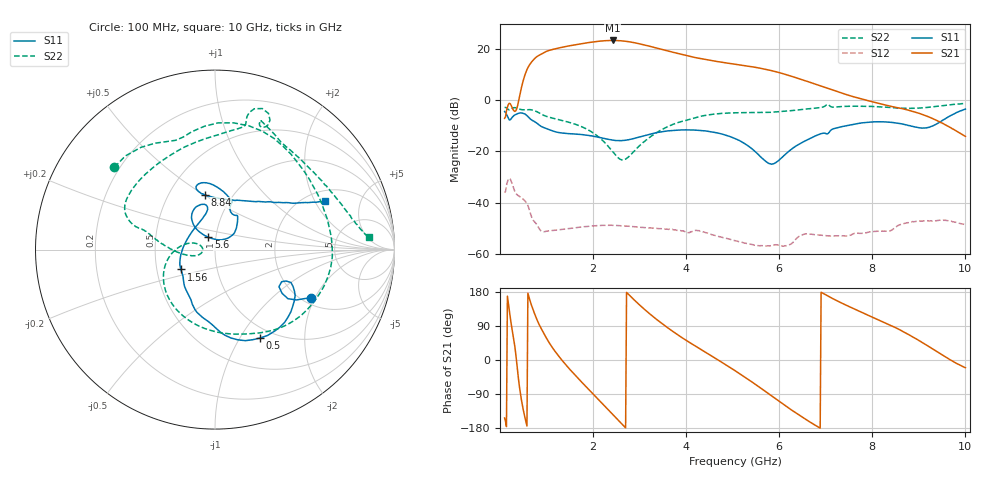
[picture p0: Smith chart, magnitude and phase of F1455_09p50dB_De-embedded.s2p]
! Integrated Device Technology
! Corporate Headquarters
! 6024 Silver Creek Valley Road
! San Jose, CA 95138  USA
! Phone:  1-408-284-8200
! Toll Free:  1-800-223-1366
! Webpage:  http://www.idt.com/
! Timing and RF Division
! 515 Groton Road, Suite 102
! Westford, MA 01886-6024
! Device:  F1455
! Description: 6-bit 0.5 dB Transmit Variable Gain Amplifier
! Frequency:  1400.0 -  2300.00 MHz
! Package:  6x6 mm Thin QFN Plastic Package: 28 pin
! State:  19
! Atten State:  9.5 dB
! Voltage:  +5.00 Volts
! Current:  217.652 mA
! Data:  The device was measured on a the F1455 evaluation board which has
!  individual transmission lines to the RF pins.  Data was collected
!  using a calibrated network analyzer.  The evaluation board was
!  de-embedded using a TRL calibration technique.
!  The reference plane is the edge of the package pin.
!  Pin  1 = CSb
!  Pin  2 = DATA
!  Pin  3 = CLK
!  Pin  4 = RSET
!  Pin  5 = GND
!  Pin  6 = RFIN  = Port 1
!  Pin  7 = GND
!  Pin  8 = NC
!  Pin  9 = NC
!  Pin 10 = NC
!  Pin 11 = NC
!  Pin 12 = NC
!  Pin 13 = NC
!  Pin 14 = /STBY
!  Pin 15 = GND
!  Pin 16 = RFOUT  = Port 2
!  Pin 17 = GND
!  Pin 18 = NC
!  Pin 19 = NC
!  Pin 20 = NC
!  Pin 21 = GND
!  Pin 22 = NC
!  Pin 23 = GND
!  Pin 24 = NC
!  Pin 25 = NC
!  Pin 26 = NC
!  Pin 27 = GND
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# GHz S dB R 50
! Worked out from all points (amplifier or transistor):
!   496 points, 100 MHz to 10 GHz, reference 50 ohm
!   highest |S21| = 23.3 dB at 2.42 GHz (marker M1)
!   |S21| within 3 dB of that: 1.25 GHz to 3.375 GHz (2.125 GHz wide, 91.9 % of centre)
!   unconditionally stable (mu >= 1): start of sweep to end of sweep
!   at 1.74 GHz: K = 10.24, MAG = 22.7 dB, |S12| = -49.6 dB
!   at 5.06 GHz: K = 36.17, MAG = 15.9 dB, |S12| = -54.9 dB
!   at 10 GHz: K = 96.42, MAG = -5.6 dB, |S12| = -48.6 dB
!   S11 on the Smith chart (normalised r, x): 100 MHz: 2.22, -1.88; 500 MHz: 0.87, -1.23; 1.56 GHz: 0.67, -0.15; 5.6 GHz: 0.92, +0.13; 8.84 GHz: 0.75, +0.50; 10 GHz: 2.46, +2.43
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0.1  -4.42 -26.7  -7.07 -152.9  -36.14 44.7  -2.80 140.7
0.38  -5.24 -39.4  -2.09 -30.2  -37.11 -111.5  -3.23 56.6
0.5  -5.15 -62.9  7.67 -130.9  -38.70 -149.6  -3.74 28.2
0.7  -7.94 -95.6  15.37 136.6  -46.45 146.9  -3.87 -18.6
0.82  -9.38 -110.7  17.33 99.4  -49.47 130.5  -4.73 -46.2
0.96  -10.83 -121.7  18.76 66.3  -51.36 124.6  -6.07 -71.1
1.26  -12.62 -139.6  20.38 10.5  -50.65 90.7  -7.59 -111.8
1.56  -13.17 -149.8  21.48 -32.7  -49.96 63.2  -9.06 -142.4
1.76  -13.42 -156.7  22.10 -58.9  -49.52 47.9  -10.39 -159.2
2.1  -14.41 -172.9  22.98 -102.1  -49.01 25.2  -14.08 175.4
2.42  -15.58 161.0  23.34 -143.4  -48.88 5.6  -20.07 162.0
2.6  -15.80 142.2  23.20 -166.5  -49.07 -4.3  -23.21 175.6
2.78  -15.39 124.6  22.81 171.0  -49.26 -13.4  -21.87 -164.7
3.08  -13.94 106.1  21.69 136.3  -49.72 -26.4  -16.45 -167.6
3.4  -12.57 100.2  20.21 103.8  -50.14 -38.6  -12.32 179.6
4.1  -11.64 110.7  17.01 44.3  -51.37 -59.3  -7.39 164.4
5.06  -15.07 131.2  14.05 -28.8  -54.91 -98.0  -4.91 149.2
5.6  -22.15 118.5  12.46 -73.9  -56.83 -101.1  -4.84 127.8
6.7  -14.63 48.7  6.74 -166.7  -52.36 -136.2  -3.23 78.7
8.36  -8.58 105.7  -2.24 93.0  -51.17 169.6  -2.82 62.7
8.84  -10.17 100.7  -4.25 62.9  -47.58 152.1  -3.19 44.5
10  -3.48 23.9  -14.14 -20.4  -48.64 80.9  -1.28 4.7
